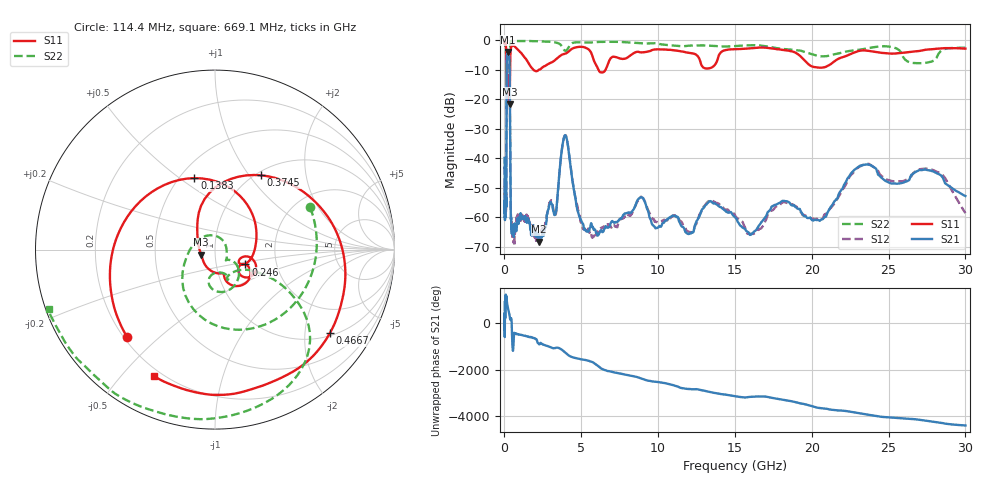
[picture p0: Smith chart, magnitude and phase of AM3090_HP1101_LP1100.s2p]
! Date/Time: Thu, Feb 28, 2019 2:08 PM
! Network Analyzer: Agilent Technologies E8364B Rev: A.07.50.67
! Sweep from 0.010 to 30.000 GHz, 1601 Points, Sweep Type: LOG
! Power Supply: 5.022 V, 0.002 A
# Hz S DB R 50
!freq MagS11 AngS11 MagS21 AngS21 MagS12 AngS12 MagS22 AngS22
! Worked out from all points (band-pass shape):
!   1601 points, 10 MHz to 30 GHz, reference 50 ohm
!   highest |S21| = -4.00 dB at 236.3 MHz (marker M1); lowest = -68.3 dB at 2.269 GHz (marker M2)
!   |S21| within 3 dB of the highest: 153.6 MHz to 324.4 MHz (170.8 MHz wide, 71.5 % of centre)
!   lowest |S11| = -21.7 dB at 333.7 MHz (marker M3), VSWR 1.18, Z = 42.8 - j2.4 ohm
!   |S11| at or under -10 dB: 144.2 MHz to 361.3 MHz (217.2 MHz wide, 85.9 % of centre); 1.866 GHz to 2.253 GHz (386.9 MHz wide, 18.8 % of centre); 6.111 GHz to 6.583 GHz (471.7 MHz wide, 7.43 % of centre)
!   |S22| runs from -23.9 to -0.1 dB; largest |S21 - S12| = 0.017
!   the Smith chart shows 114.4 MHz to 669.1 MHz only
!   S11 on the Smith chart (normalised r, x): 114.4 MHz: 0.21, -0.40; 138.3 MHz: 0.59, +0.57; 246 MHz: 1.38, -0.24; 374.5 MHz: 1.06, +1.15; 466.7 MHz: 1.08, -2.69; 669.1 MHz: 0.17, -0.62
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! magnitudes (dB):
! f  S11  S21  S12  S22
! 10 MHz  -0.3  -39.9  -43.5  -0.6
! 38.04 MHz  -0.4  -58.4  -58.4  -1.4
! 114.4 MHz  -3.2  -56.5  -53.5  -4.7
! 138.3 MHz  -7.7  -19.4  -19.4  -9.1
! 144.7 MHz  -10.2  -11.7  -11.7  -18.1
! 236.3 MHz  -15.7  -4.0  -4.0  -16.9
! 246 MHz  -14.5  -4.0  -4.0  -17.8
! 333.7 MHz  -21.7  -8.7  -8.7  -9.6
! 374.5 MHz  -6.2  -37.8  -37.8  -1.3
! 409.7 MHz  -3.2  -58.4  -57.1  -0.5
! 466.7 MHz  -2.0  -64.1  -61.7  -0.3
! 550.5 MHz  -1.9  -64.6  -65.0  -0.2
! 669.1 MHz  -2.1  -62.9  -64.7  -0.1
! 2.084 GHz  -10.5  -65.5  -67.9  -0.4
! 2.269 GHz  -10.0  -68.3  -66.5  -0.4
! 3.318 GHz  -6.7  -58.8  -59.5  -0.8
! 3.934 GHz  -4.6  -32.3  -32.2  -3.6
! 5.154 GHz  -2.4  -63.3  -64.2  -0.8
! 7.926 GHz  -6.1  -58.6  -59.6  -0.7
! 16.29 GHz  -2.6  -64.7  -65.3  -1.7
! 23.48 GHz  -3.5  -42.2  -42.0  -2.9
! 30 GHz  -2.9  -52.8  -58.6  -2.6
